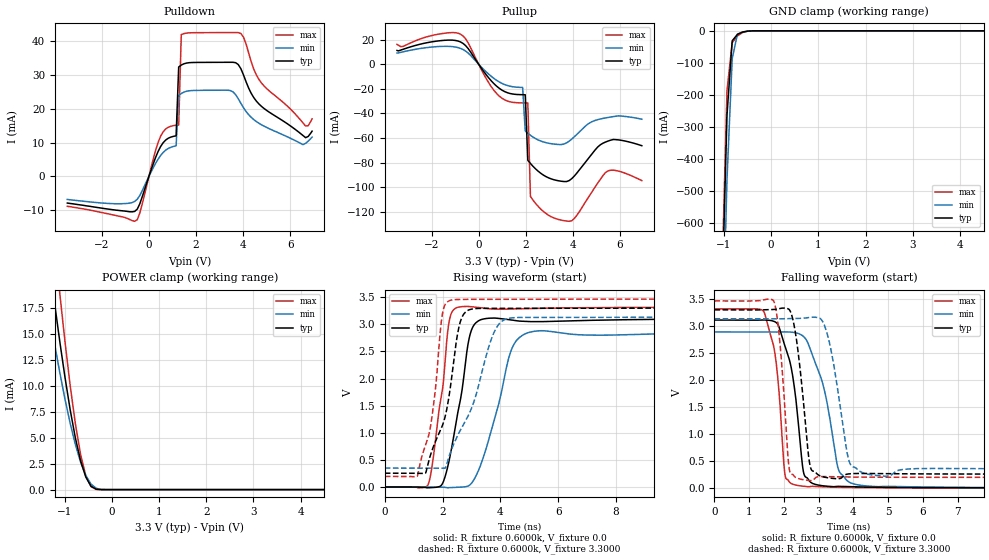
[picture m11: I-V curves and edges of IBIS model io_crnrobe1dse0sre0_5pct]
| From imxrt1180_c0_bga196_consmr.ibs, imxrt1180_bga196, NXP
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[Model]  io_crnrobe1dse0sre0_5pct
|   Model io_crnrobe1dse0sre0_5pct
| This model was characterised for following simulation conditions:
| External (pad) voltage:
|   - Typ: 3.3V,   - Min: 3.135V,   - Max: 3.465V
| Library cells for typ/min/max conditions are connected as defined below:
|  PAD_IO - External Pad
|  ipp_do - Core Input
|  ipp_obe - Output Buffer Enable
|  ASRCN3V3[3] - NC
|  ASRCN3V3[4] - NC
|  ASRCP3V3[4] - NC
|  REFAPBIAS3V3 - gnde
|  REFBAMPL3V3 - vdd1v8
|  REFCAMPH3V3 - vdd1v8
|  REFDNBIAS3V3 - vdd1v8
|  REFH3V3 - REFH3V3
|  REFL3V3 - REFL3V3
|  gnde - gnde
|  ipp_dse - gnde
|  ipp_ina235_3v - NC
|  ipp_ina40_3v - NC
|  ipp_ina_mux - NC
|  ipp_ind - NC
|  ipp_ind_1p8v - NC
|  ipp_ind_3v - NC
|  ipp_sre - gnde
|  vdd - vdd
|  vdd1v8 - vdd1v8
|  vdda - vdde3v3
|  vdde3v3 - vdde3v3
| All other pins connected to ground
Model_type I/O
Polarity   Non-Inverting
Enable   Active-High
Vinl =   0.9900V
Vinh =   2.3100V
Vmeas =  1.6500V
Cref =   15.0000pF
Rref =   0.6000k
Vref =   0.0V
C_comp   4.0038pF   3.8208pF   4.1241pF
|C_comp_pullup   0.5150pF   0.5903pF   0.4959pF
|C_comp_pulldown   2.0816pF   2.1812pF   1.8614pF
[Model Spec]
| variable   typ   min   max
Vinh   2.3100V   NA   NA
Vinl   0.9900V   NA   NA
Vref   0.0V   0.0V   0.0V
Cref   15.0000pF   15.0000pF   15.0000pF
Rref   0.6000k   0.6000k   0.6000k
[Receiver Thresholds]
Vcross_high  =   0.0V
Vcross_low  =   0.0V
Vdiff_ac  =   0.0V
Vdiff_dc  =   0.0V
Tdiffslew_ac  =   0.0S
[Temperature Range]   25.0000   0.1250k   -40.0000
[Voltage Range]   3.3000V   3.1350V   3.4650V
[Pullup Reference]   3.3000V   3.1350V   3.4650V
[Pulldown Reference]   0.0V   0.0V   0.0V
[POWER Clamp Reference]   3.3000V   3.1350V   3.4650V
[GND Clamp Reference]   0.0V   0.0V   0.0V
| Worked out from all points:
|   slope of the pulldown table from 0 to 0.495 V, typ, clamps not added: 56 ohm
|   slope of the pullup table from 0 to 0.495 V, typ, clamps not added: 39.3 ohm
|   GND clamp passes 1 mA (typ) near -0.50 V on its own axis
|   POWER clamp passes 1 mA (typ) near -0.52 V on its own axis
|   rising waveform, R_fixture 0.6000k, V_fixture 0.0: 20-80 % time 560ps typ, 826ps min, 428ps max; typ from 0 V to 3.11 V
|   rising waveform, R_fixture 0.6000k, V_fixture 3.3000: 20-80 % time 705ps typ, 1.11ns min, 450ps max; typ from 0.254 V to 3.3 V
|   falling waveform, R_fixture 0.6000k, V_fixture 0.0: 20-80 % time 397ps typ, 587ps min, 280ps max; typ from 3.11 V to 0 V
|   falling waveform, R_fixture 0.6000k, V_fixture 3.3000: 20-80 % time 292ps typ, 406ps min, 220ps max; typ from 3.3 V to 0.254 V
[Pulldown]
|Voltage   I(typ)   I(min)   I(max)
-3.465V   -7.9mA     -6.83mA    -8.86mA
-495mV    -9.702mA   -6.763mA   -12.83mA
495mV     8.834mA    6.188mA    11.88mA
1.155V    12.02mA    9.055mA    15.17mA
1.265V    32.44mA    23.98mA    15.25mA
1.375V    33.01mA    24.57mA    42.05mA
1.485V    33.37mA    24.97mA    42.33mA
3.465V    33.83mA    25.43mA    42.63mA
3.905V    31.93mA    21.67mA    42.36mA
4.785V    20.73mA    15.29mA    27.65mA
6.655V    11.48mA    9.805mA    14.92mA
6.93V     13.41mA    11.66mA    17.06mA
[Pullup]
|Voltage   I(typ)   I(min)   I(max)
-3.465V   11.16mA    9.087mA    16.08mA
-1.21V    19.58mA    14.42mA    25.6mA
-550mV    15.05mA    10.64mA    20.55mA
770mV     -17.95mA   -13.16mA   -23.93mA
1.87V     -24.79mA   -18.89mA   -31.45mA
1.98V     -24.83mA   -54.24mA   -31.49mA
2.09V     -78.09mA   -56.07mA   -31.51mA
2.2V      -80.61mA   -57.72mA   -107.4mA
3.08V     -93.14mA   -64.56mA   -123.9mA
3.96V     -92.86mA   -60.73mA   -127.1mA
5.5V      -62.41mA   -43.25mA   -86.61mA
6.93V     -66.2mA    -44.66mA   -94.52mA
[GND_clamp]
|Voltage   I(typ)   I(min)   I(max)
-3.465V   -18.65A    -18.54A    -19.59A
-1.045V   -856.4mA   -1.07A     -789.2mA
-935mV    -262.9mA   -462.2mA   -186.4mA
-825mV    -31.14mA   -87.01mA   -37.16mA
-715mV    -11.21mA   -10.51mA   -15.88mA
-605mV    -3.859mA   -3.519mA   -5.394mA
-385mV    -79.67uA   -219.6uA   -43.93uA
6.93V     0A         0A         0A
[POWER_clamp]
|Voltage   I(typ)   I(min)   I(max)
-3.465V   98.91mA    78.43mA    126mA
-1.43V    25.78mA    19.9mA     34.19mA
-1.32V    21.78mA    16.89mA    28.92mA
-1.21V    17.92mA    14mA       23.79mA
-1.1V     14.24mA    11.26mA    18.86mA
-880mV    7.673mA    6.373mA    9.998mA
-770mV    4.965mA    4.333mA    6.33mA
-660mV    2.777mA    2.644mA    3.379mA
-550mV    1.212mA    1.363mA    1.332mA
-440mV    333.5uA    531.5uA    282.6uA
-330mV    37.61uA    130.9uA    15.04uA
6.93V     0A         0A         0A
[Ramp]
| variable   typ   min   max
dV/dt_r  1.8668/0.5597n   1.7341/0.8261n   1.9910/0.4284n
dV/dt_f  1.8274/0.2918n   1.6719/0.4058n   1.9622/0.2201n
R_load = 0.6000k
[Rising Waveform]
R_fixture= 0.6000k
V_fixture= 0.0
V_fixture_min= 0.0
V_fixture_max= 0.0
|time   V(typ)   V(min)   V(max)
0s        139.9nV    3.48uV     63.01nV
1.502ns   -14.33mV   -963.7uV   46.76mV
1.996ns   62.43mV    -3.934mV   1.797V
2.229ns   494.4mV    -12.17mV   3.058V
2.663ns   1.754V     -2.784mV   3.326V
2.91ns    2.72V      24.76mV    3.329V
3.145ns   3.025V     192.8mV    3.317V
4.403ns   3.077V     2.56V      3.283V
5.282ns   3.049V     2.878V     3.295V
60ns      3.111V     2.89V      3.318V
[Rising Waveform]
R_fixture= 0.6000k
V_fixture= 3.3000
V_fixture_min= 3.1350
V_fixture_max= 3.4650
|time   V(typ)   V(min)   V(max)
0s        254.3mV    348.5mV    194.7mV
1.126ns   253.7mV    348.4mV    197.9mV
1.589ns   603.1mV    348.4mV    1.137V
2.009ns   1.155V     345.9mV    3.233V
2.414ns   2.453V     828mV      3.456V
2.607ns   3.037V     1.039V     3.459V
2.832ns   3.243V     1.259V     3.461V
3.782ns   3.295V     2.854V     3.461V
4.467ns   3.295V     3.123V     3.461V
60ns      3.3V       3.135V     3.465V
[Falling Waveform]
R_fixture= 0.6000k
V_fixture= 0.0
V_fixture_min= 0.0
V_fixture_max= 0.0
|time   V(typ)   V(min)   V(max)
0s        3.111V     2.89V      3.318V
1.406ns   3.112V     2.89V      3.28V
1.828ns   3.025V     2.888V     1.999V
2.048ns   2.59V      2.892V     189.3mV
2.547ns   350.1mV    2.815V     30.66mV
2.66ns    188.7mV    2.725V     22.31mV
3.146ns   36.47mV    1.86V      18.18mV
3.599ns   27.68mV    293.6mV    9.353mV
4.445ns   13.17mV    32.15mV    3.274mV
60ns      2.412uV    3.897uV    2.125uV
[Falling Waveform]
R_fixture= 0.6000k
V_fixture= 3.3000
V_fixture_min= 3.1350
V_fixture_max= 3.4650
|time   V(typ)   V(min)   V(max)
0s        3.3V       3.135V     3.465V
1.714ns   3.307V     3.135V     3.451V
1.882ns   3.326V     3.134V     2.704V
2.168ns   3.291V     3.138V     301.2mV
2.392ns   2.602V     3.141V     177.3mV
2.752ns   412.4mV    3.16V      134.7mV
3.249ns   188.1mV    2.847V     208.3mV
3.889ns   260.3mV    470.9mV    201mV
4.814ns   263.6mV    220.1mV    196.9mV
60ns      254.3mV    348.5mV    194.7mV
